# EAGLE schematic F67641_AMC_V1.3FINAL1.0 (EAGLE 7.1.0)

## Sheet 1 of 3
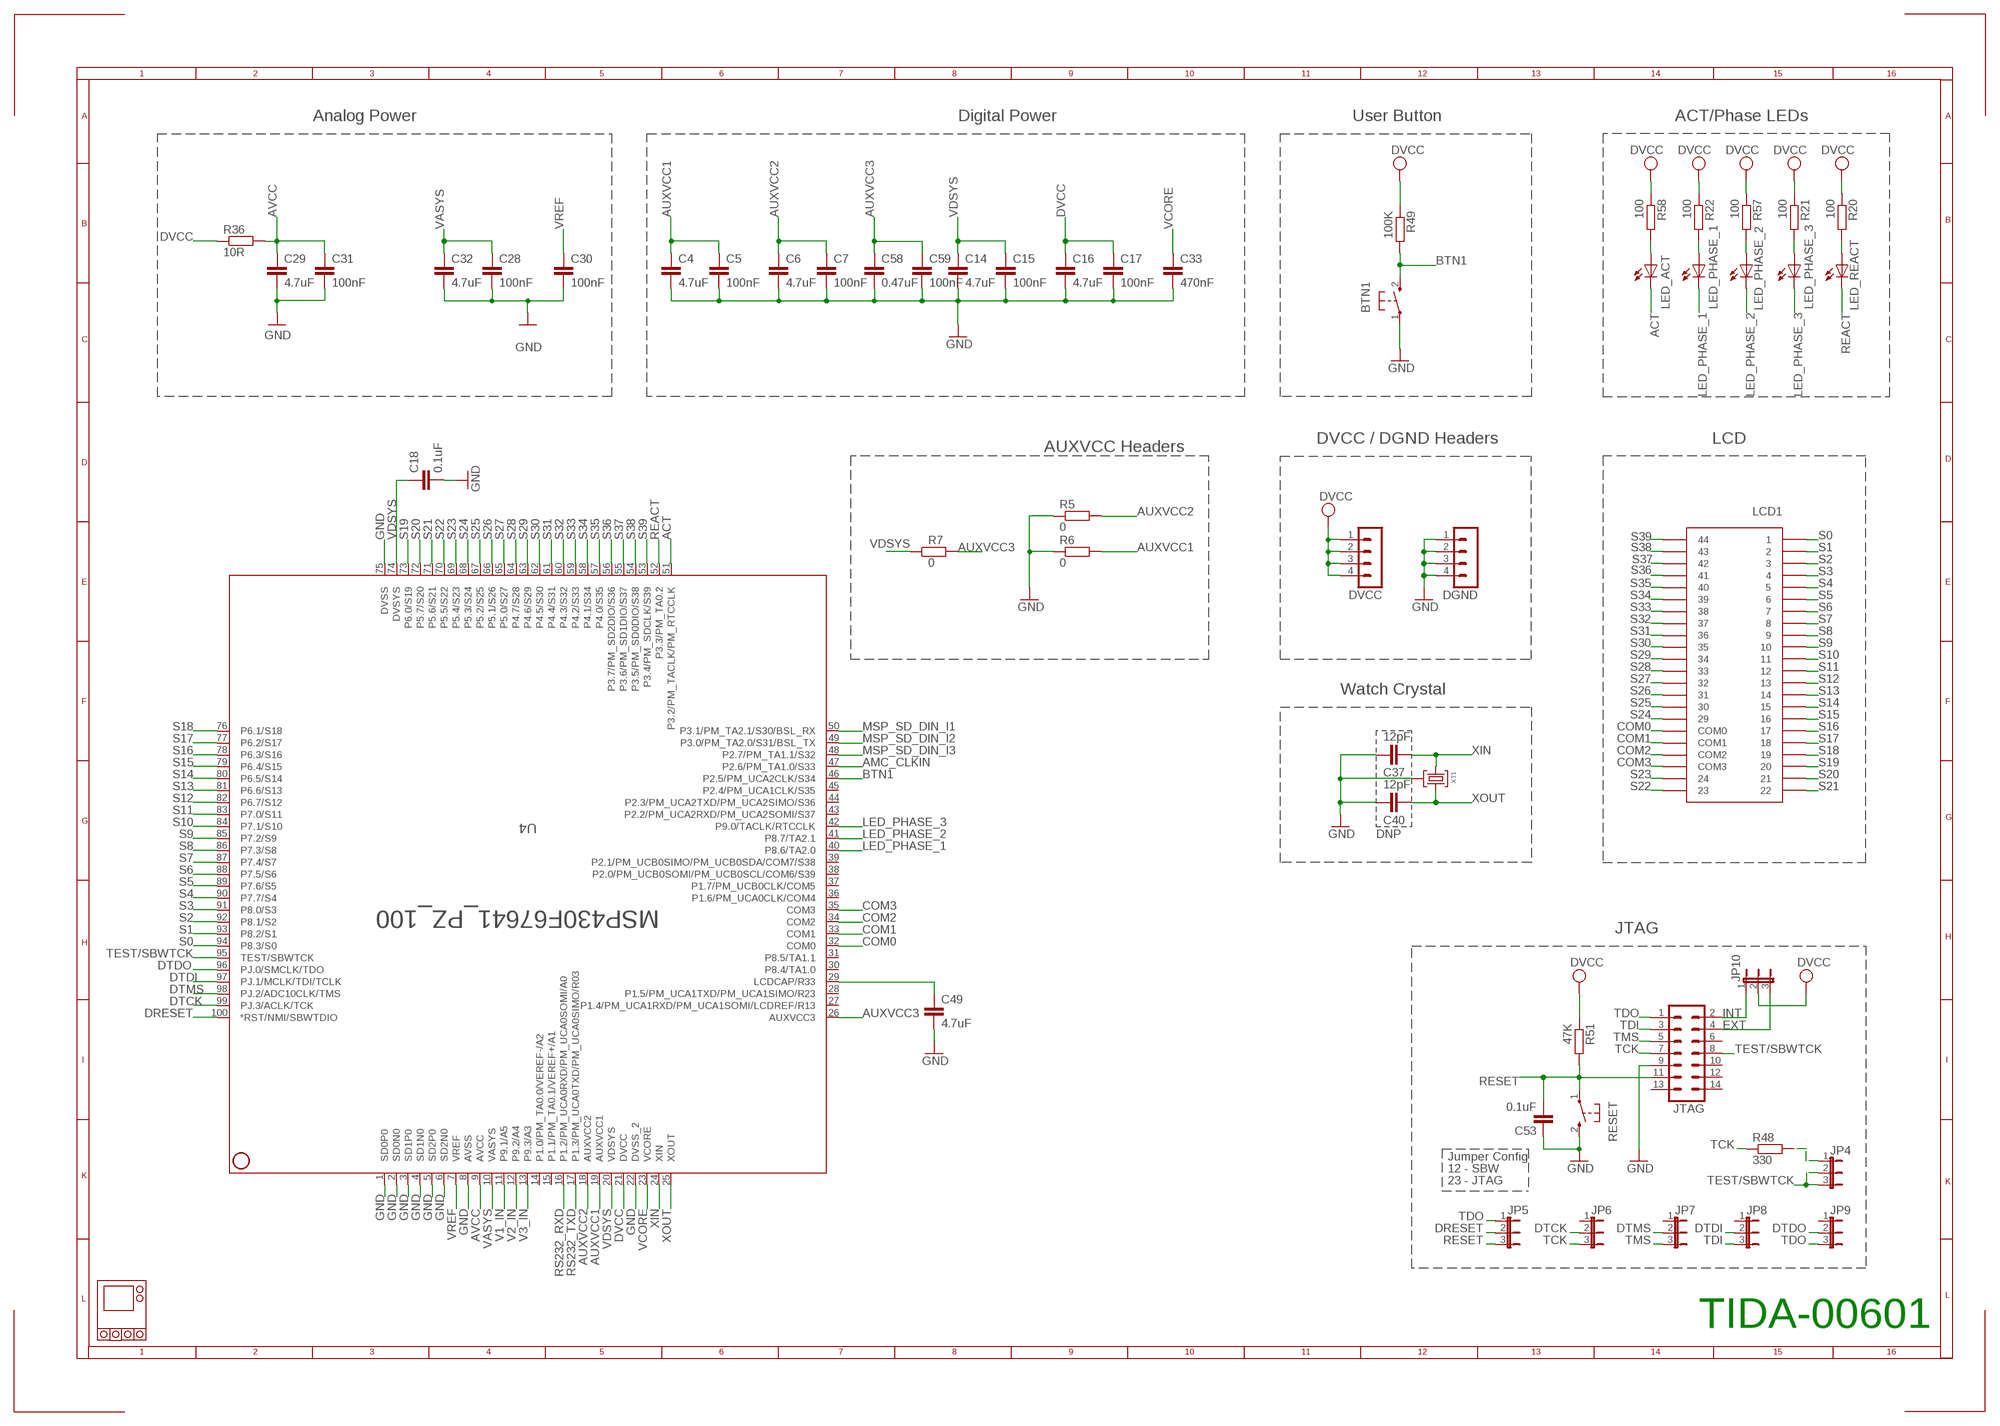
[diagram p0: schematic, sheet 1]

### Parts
BTN1  PB  [PBTH]
C4  4.7uF  C-EUC0603  [C0603]
C5  100nF  C-EUC0603  [C0603]
C6  4.7uF  C-EUC0603  [C0603]
C7  100nF  C-EUC0603  [C0603]
C14  4.7uF  C-EUC0603  [C0603]
C15  100nF  C-EUC0603  [C0603]
C16  4.7uF  C-EUC0603  [C0603]
C17  100nF  C-EUC0603  [C0603]
C18  0.1uF  C-EUC0603  [C0603]
C28  100nF  C-EUC0603  [C0603]
C29  4.7uF  C-EUC0603  [C0603]
C30  100nF  C-EUC0603  [C0603]
C31  100nF  C-EUC0603  [C0603]
C32  4.7uF  C-EUC0603  [C0603]
C33  470nF  C-EUC0603  [C0603]
C37  12pF  C-EUC0603  [C0603]
C40  12pF  C-EUC0603  [C0603]
C49  4.7uF  C-EUC0603  [C0603]
C53  0.1uF  C-EUC0603  [C0603]
C58  0.47uF  C-EUC0603  [C0603]
C59  100nF  C-EUC0603  [C0603]
CASE1  3_PHASE_CASE  [3_PHASE_CASE]
DGND  MA04-1  [MA04-1]
DVCC  MA04-1  [MA04-1]
JP4  JP2E  [JP2]
JP5  JP2E  [JP2]
JP6  JP2E  [JP2]
JP7  JP2E  [JP2]
JP8  JP2E  [JP2]
JP9  JP2E  [JP2]
JP10  JP2E  [JP2]
JTAG  ML14  [ML14]
LCD1  TI_160SEG_LCD  [TI_160SEG_LCD]
LED_ACT  LED3MM  [LED3MM]
LED_PHASE_1  LED3MM  [LED3MM]
LED_PHASE_2  LED3MM  [LED3MM]
LED_PHASE_3  LED3MM  [LED3MM]
LED_REACT  LED3MM  [LED3MM]
R5  0  R-EU_R0603  [R0603]
R6  0  R-EU_R0603  [R0603]
R7  0  R-EU_R0603  [R0603]
R20  100  R-EU_R0603  [R0603]
R21  100  R-EU_R0603  [R0603]
R22  100  R-EU_R0603  [R0603]
R36  10R  R-EU_R0805  [R0805]
R48  330  R-EU_R0603  [R0603]
R49  100K  R-EU_R0603  [R0603]
R51  47K  R-EU_R0603  [R0603]
R57  100  R-EU_R0603  [R0603]
R58  100  R-EU_R0603  [R0603]
RESET  PB  [PBTH]
U4  MSP430F67641_PZ_100  [PZ100]
XT1  CM200T  [CM200T]

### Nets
ACT: LED_ACT.K(C) U4.51(P3.2/PM_TACLK/PM_RTCCLK) ; also sheet 2
AMC_CLKIN: U4.47(P2.6/PM_TA1.0/S33) ; also sheet 3
AUXVCC1: C4.1 C5.1 R6.2 U4.19(AUXVCC1)
AUXVCC2: C6.1 C7.1 R5.2 U4.18(AUXVCC2)
AUXVCC3: C58.1 C59.1 R7.2 U4.26(AUXVCC3)
AVCC: C29.1 C31.1 R36.2 U4.9(AVCC) ; also sheet 2
BTN1: BTN1.2(S) R49.2 U4.46(P2.5/PM_UCA2CLK/S34)
COM0: LCD1.COM0 U4.32(COM0)
COM1: LCD1.COM1 U4.33(COM1)
COM2: LCD1.COM2 U4.34(COM2)
COM3: LCD1.COM3 U4.35(COM3)
DRESET: JP5.2 U4.100(*RST/NMI/SBWTDIO)
DTCK: JP6.2 U4.99(PJ.3/ACLK/TCK)
DTDI: JP8.2 U4.97(PJ.1/MCLK/TDI/TCLK)
DTDO: JP9.2 U4.96(PJ.0/SMCLK/TDO)
DTMS: JP7.2 U4.98(PJ.2/ADC10CLK/TMS)
DVCC: C16.1 C17.1 DVCC.1 DVCC.2 DVCC.3 DVCC.4 JP10.2 R20.1 R21.1 R22.1 R36.1 R49.1 R51.1 R57.1 R58.1 U4.21(DVCC) ; also sheet 2,3
EXT: JP10.3 JTAG.4
GND: BTN1.1(P) C4.2 C5.2 C6.2 C7.2 C14.2 C15.2 C16.2 C17.2 C18.2 C28.2 C29.2 C30.2 C31.2 C32.2 C33.2 C37.2 C40.2 C49.2 C53.1 C58.2 C59.2 DGND.1 DGND.2 DGND.3 DGND.4 JTAG.9 R5.1 R6.1 RESET.2(S) U4.1(SD0P0) U4.2(SD0N0) U4.3(SD1P0) U4.4(SD1N0) U4.5(SD2P0) U4.6(SD2N0) U4.8(AVSS) U4.22(DVSS_2) U4.75(DVSS) XT1.P3 ; also sheet 2,3
INT: JP10.1 JTAG.2
LED_PHASE_1: LED_PHASE_1.K(C) U4.40(P8.6/TA2.0)
LED_PHASE_2: LED_PHASE_2.K(C) U4.41(P8.7/TA2.1)
LED_PHASE_3: LED_PHASE_3.K(C) U4.42(P9.0/TACLK/RTCCLK)
MSP_SD_DIN_I1: U4.50(P3.1/PM_TA2.1/S30/BSL_RX) ; also sheet 3
MSP_SD_DIN_I2: U4.49(P3.0/PM_TA2.0/S31/BSL_TX) ; also sheet 3
MSP_SD_DIN_I3: U4.48(P2.7/PM_TA1.1/S32) ; also sheet 3
N$4: C49.1 U4.29(LCDCAP/R33)
N$5: LED_REACT.A R20.2
N$6: LED_PHASE_3.A R21.2
N$7: LED_PHASE_1.A R22.2
N$34: JP4.1 R48.2
N$44: LED_ACT.A R58.2
N$46: LED_PHASE_2.A R57.2
REACT: LED_REACT.K(C) U4.52(P3.3/PM_TA0.2) ; also sheet 2
RESET: C53.2 JP5.3 JTAG.11 R51.2 RESET.1(P)
RS232_RXD: U4.16(P1.2/PM_UCA0RXD/PM_UCA0SOMI/A0) ; also sheet 2
RS232_TXD: U4.17(P1.3/PM_UCA0TXD/PM_UCA0SIMO/R03) ; also sheet 2
S0: LCD1.1 U4.94(P8.3/S0)
S1: LCD1.2 U4.93(P8.2/S1)
S2: LCD1.3 U4.92(P8.1/S2)
S3: LCD1.4 U4.91(P8.0/S3)
S4: LCD1.5 U4.90(P7.7/S4)
S5: LCD1.6 U4.89(P7.6/S5)
S6: LCD1.7 U4.88(P7.5/S6)
S7: LCD1.8 U4.87(P7.4/S7)
S8: LCD1.9 U4.86(P7.3/S8)
S9: LCD1.10 U4.85(P7.2/S9)
S10: LCD1.11 U4.84(P7.1/S10)
S11: LCD1.12 U4.83(P7.0/S11)
S12: LCD1.13 U4.82(P6.7/S12)
S13: LCD1.14 U4.81(P6.6/S13)
S14: LCD1.15 U4.80(P6.5/S14)
S15: LCD1.16 U4.79(P6.4/S15)
S16: LCD1.17 U4.78(P6.3/S16)
S17: LCD1.18 U4.77(P6.2/S17)
S18: LCD1.19 U4.76(P6.1/S18)
S19: LCD1.20 U4.73(P6.0/S19)
S20: LCD1.21 U4.72(P5.7/S20)
S21: LCD1.22 U4.71(P5.6/S21)
S22: LCD1.23 U4.70(P5.5/S22)
S23: LCD1.24 U4.69(P5.4/S23)
S24: LCD1.29 U4.68(P5.3/S24)
S25: LCD1.30 U4.67(P5.2/S25)
S26: LCD1.31 U4.66(P5.1/S26)
S27: LCD1.32 U4.65(P5.0/S27)
S28: LCD1.33 U4.64(P4.7/S28)
S29: LCD1.34 U4.63(P4.6/S29)
S30: LCD1.35 U4.62(P4.5/S30)
S31: LCD1.36 U4.61(P4.4/S31)
S32: LCD1.37 U4.60(P4.3/S32)
S33: LCD1.38 U4.59(P4.2/S33)
S34: LCD1.39 U4.58(P4.1/S34)
S35: LCD1.40 U4.57(P4.0/S35)
S36: LCD1.41 U4.56(P3.7/PM_SD2DIO/S36)
S37: LCD1.42 U4.55(P3.6/PM_SD1DIO/S37)
S38: LCD1.43 U4.54(P3.5/PM_SD0DIO/S38)
S39: LCD1.44 U4.53(P3.4/PM_SDCLK/S39)
TCK: JP6.3 JTAG.7 R48.1
TDI: JP8.3 JTAG.3
TDO: JP5.1 JP9.3 JTAG.1
TEST/SBWTCK: JP4.2 JP4.3 JTAG.8 U4.95(TEST/SBWTCK)
TMS: JP7.3 JTAG.5
V1_IN: U4.11(P9.1/A5) ; also sheet 2
V2_IN: U4.12(P9.2/A4) ; also sheet 2
V3_IN: U4.13(P9.3/A3) ; also sheet 2
VASYS: C28.1 C32.1 U4.10(VASYS)
VCORE: C33.1 U4.23(VCORE)
VDSYS: C14.1 C15.1 C18.1 R7.1 U4.20(VDSYS) U4.74(DVSYS)
VREF: C30.1 U4.7(VREF)
XIN: C37.1 U4.24(XIN) XT1.P2
XOUT: C40.1 U4.25(XOUT) XT1.P1
Unconnected: JP6.1 JP7.1 JP8.1 JP9.1 JTAG.6 JTAG.10 JTAG.12 JTAG.13 JTAG.14 U4.14(P1.0/PM_TA0.0/VEREF-/A2) U4.15(P1.1/PM_TA0.1/VEREF+/A1) U4.27(P1.4/PM_UCA1RXD/PM_UCA1SOMI/LCDREF/R13) U4.28(P1.5/PM_UCA1TXD/PM_UCA1SIMO/R23) U4.30(P8.4/TA1.0) U4.31(P8.5/TA1.1) U4.36(P1.6/PM_UCA0CLK/COM4) U4.37(P1.7/PM_UCB0CLK/COM5) U4.38(P2.0/PM_UCB0SOMI/PM_UCB0SCL/COM6/S39) U4.39(P2.1/PM_UCB0SIMO/PM_UCB0SDA/COM7/S38) U4.43(P2.2/PM_UCA2RXD/PM_UCA2SOMI/S37) U4.44(P2.3/PM_UCA2TXD/PM_UCA2SIMO/S36) U4.45(P2.4/PM_UCA1CLK/S35)

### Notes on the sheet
- Analog Power | Digital Power | User Button | ACT/Phase LEDs
- DVCC / DGND Headers | LCD
- AUXVCC Headers
- Watch Crystal
- DNP
- JTAG
- Jumper Config
- 12 - SBW
- 23 - JTAG
- TIDA-00601

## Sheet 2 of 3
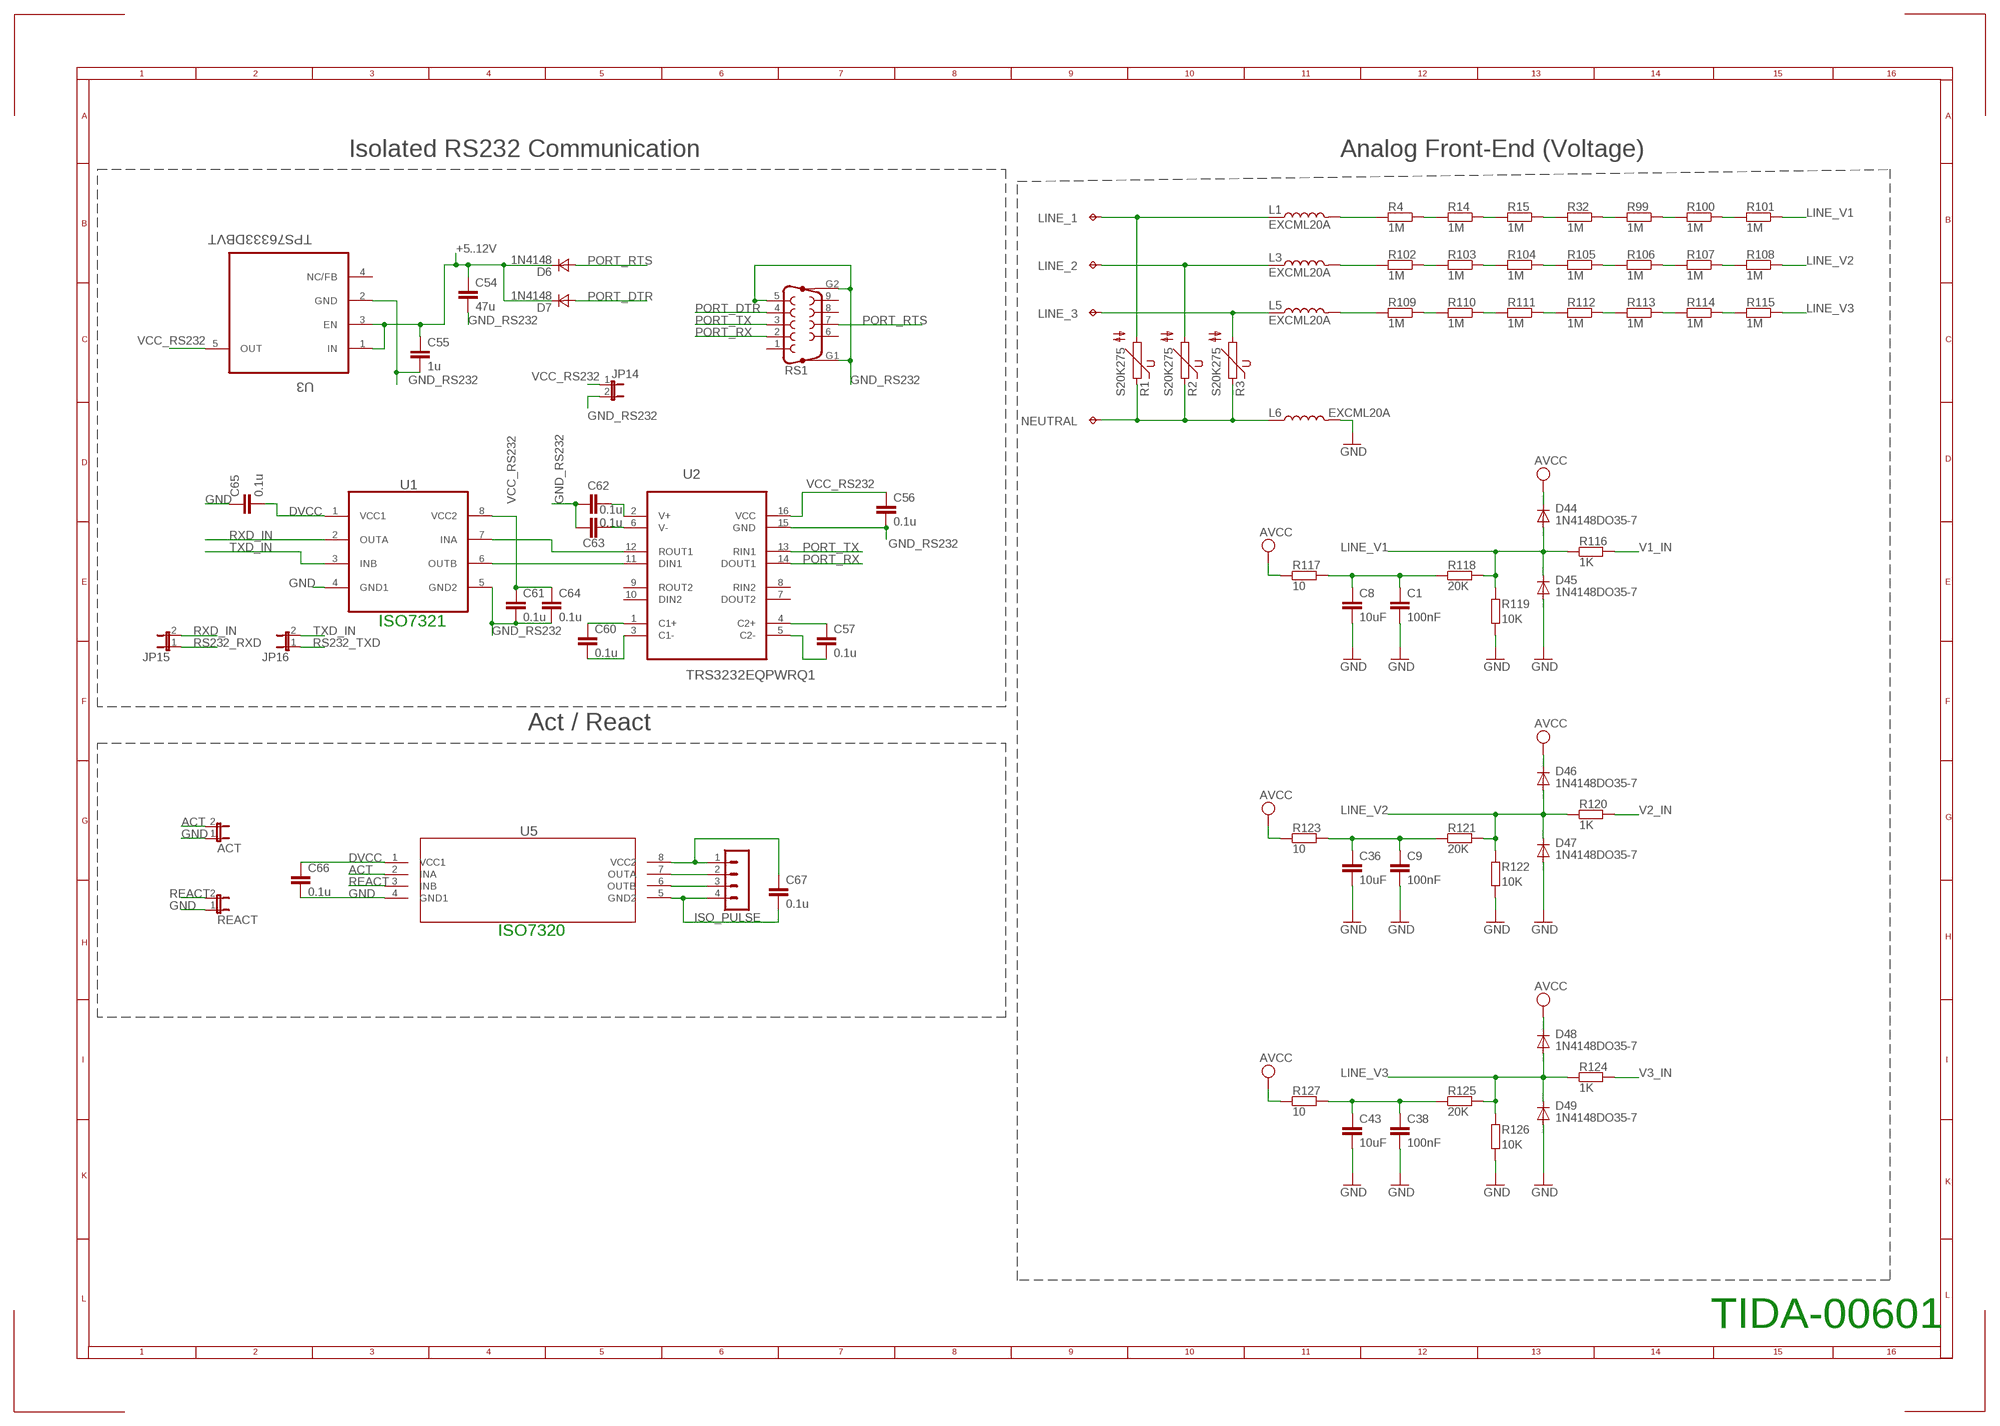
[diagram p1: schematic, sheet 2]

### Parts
ACT  JP1E  [JP1]
C1  100nF  C-EUC0805  [C0805]
C8  10uF  C-EUC0805  [C0805]
C9  100nF  C-EUC0805  [C0805]
C36  10uF  C-EUC0805  [C0805]
C38  100nF  C-EUC0805  [C0805]
C43  10uF  C-EUC0805  [C0805]
C54  47u  C-EUC1206K  [C1206K]
C55  1u  C-EUC0603  [C0603]
C56  0.1u  C-EUC0603  [C0603]
C57  0.1u  C-EUC0603  [C0603]
C60  0.1u  C-EUC0603  [C0603]
C61  0.1u  C-EUC0603  [C0603]
C62  0.1u  C-EUC0603  [C0603]
C63  0.1u  C-EUC0603  [C0603]
C64  0.1u  C-EUC0603  [C0603]
C65  0.1u  C-EUC0603  [C0603]
C66  0.1u  C-EUC0603  [C0603]
C67  0.1u  C-EUC0603  [C0603]
D6  1N4148  DSOD323  [SOD323]
D7  1N4148  DSOD323  [SOD323]
D44  1N4148DO35-7  DIODE-SOD523  [SOD523]
D45  1N4148DO35-7  DIODE-SOD523  [SOD523]
D46  1N4148DO35-7  DIODE-SOD523  [SOD523]
D47  1N4148DO35-7  DIODE-SOD523  [SOD523]
D48  1N4148DO35-7  DIODE-SOD523  [SOD523]
D49  1N4148DO35-7  DIODE-SOD523  [SOD523]
ISO_PULSE  MA04-1  [MA04-1]
JP14  JP1E  [JP1]
JP15  JP1E  [JP1]
JP16  JP1E  [JP1]
L1  EXCML20A  EXCELSA390805  [R0805]
L3  EXCML20A  EXCELSA390805  [R0805]
L5  EXCML20A  EXCELSA390805  [R0805]
L6  EXCML20A  EXCELSA390805  [R0805]
LINE_1  TPPAD1-20  [P1-20]
LINE_2  TPPAD1-20  [P1-20]
LINE_3  TPPAD1-20  [P1-20]
NEUTRAL  TPPAD1-20  [P1-20]
R1  S20K275  [S20K275]
R2  S20K275  [S20K275]
R3  S20K275  [S20K275]
R4  1M  R-EU_R0805  [R0805]
R14  1M  R-EU_R0805  [R0805]
R15  1M  R-EU_R0805  [R0805]
R32  1M  R-EU_R0805  [R0805]
R99  1M  R-EU_R0805  [R0805]
R100  1M  R-EU_R0805  [R0805]
R101  1M  R-EU_R0805  [R0805]
R102  1M  R-EU_R0805  [R0805]
R103  1M  R-EU_R0805  [R0805]
R104  1M  R-EU_R0805  [R0805]
R105  1M  R-EU_R0805  [R0805]
R106  1M  R-EU_R0805  [R0805]
R107  1M  R-EU_R0805  [R0805]
R108  1M  R-EU_R0805  [R0805]
R109  1M  R-EU_R0805  [R0805]
R110  1M  R-EU_R0805  [R0805]
R111  1M  R-EU_R0805  [R0805]
R112  1M  R-EU_R0805  [R0805]
R113  1M  R-EU_R0805  [R0805]
R114  1M  R-EU_R0805  [R0805]
R115  1M  R-EU_R0805  [R0805]
R116  1K  R-EU_R0805  [R0805]
R117  10  R-EU_R0805  [R0805]
R118  20K  R-EU_R0805  [R0805]
R119  10K  R-EU_R0805  [R0805]
R120  1K  R-EU_R0805  [R0805]
R121  20K  R-EU_R0805  [R0805]
R122  10K  R-EU_R0805  [R0805]
R123  10  R-EU_R0805  [R0805]
R124  1K  R-EU_R0805  [R0805]
R125  20K  R-EU_R0805  [R0805]
R126  10K  R-EU_R0805  [R0805]
R127  10  R-EU_R0805  [R0805]
REACT  JP1E  [JP1]
RS1  F09VP  [F09VP]
U1  ISO7421D  [SOIC127P600X175-8N]
U2  TRS3232EQPWRQ1  [SOP65P640X120-16N]
U3  TPS76333DBVT  [SOT95P280X145-5N]
U5  ISO7420_D_8  [D8]

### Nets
+5..12V: C54.1 C55.1 D6.1(C) D7.1(C) U3.1(IN) U3.3(EN)
ACT: ACT.2 U5.2(INA) ; also sheet 1
AVCC: D44.C D46.C D48.C R117.1 R123.1 R127.1 ; also sheet 1
DVCC: C65.2 C66.1 U1.1(VCC1) U5.1(VCC1) ; also sheet 1,3
GND: ACT.1 C1.2 C8.2 C9.2 C36.2 C38.2 C43.2 C65.1 C66.2 D45.A D47.A D49.A L6.2 R119.1 R122.1 R126.1 REACT.1 U1.4(GND1) U5.4(GND1) ; also sheet 1,3
GND_RS232: C54.2 C55.2 C56.2 C61.2 C62.1 C63.1 C64.2 JP14.2 RS1.5 RS1.G1 RS1.G2 U1.5(GND2) U2.15(GND) U3.2(GND)
LINE_1: L1.1 LINE_1.TP R1.2
LINE_2: L3.1 LINE_2.TP R2.2
LINE_3: L5.1 LINE_3.TP R3.2
LINE_V1: D44.A D45.C R101.1 R116.1 R118.2 R119.2
LINE_V2: D46.A D47.C R108.1 R120.1 R121.2 R122.2
LINE_V3: D48.A D49.C R115.1 R124.1 R125.2 R126.2
N$3: C67.1 ISO_PULSE.1 U5.8(VCC2)
N$9: C57.1 U2.4(C2+)
N$11: ISO_PULSE.2 U5.7(OUTA)
N$12: ISO_PULSE.3 U5.6(OUTB)
N$22: C57.2 U2.5(C2-)
N$24: C60.1 U2.1(C1+)
N$26: C60.2 U2.3(C1-)
N$28: U1.7(INA) U2.12(ROUT1)
N$33: U1.6(OUTB) U2.11(DIN1)
N$36: C62.2 U2.2(V+)
N$40: C63.2 U2.6(V-)
N$43: C67.2 ISO_PULSE.4 U5.5(GND2)
N$96: R4.1 R14.2
N$97: R14.1 R15.2
N$98: R15.1 R32.2
N$99: R32.1 R99.2
N$100: R99.1 R100.2
N$101: R100.1 R101.2
N$102: R102.1 R103.2
N$103: R103.1 R104.2
N$104: R104.1 R105.2
N$105: R105.1 R106.2
N$106: R106.1 R107.2
N$107: R107.1 R108.2
N$108: R109.1 R110.2
N$109: R110.1 R111.2
N$110: R111.1 R112.2
N$111: R112.1 R113.2
N$112: R113.1 R114.2
N$113: R114.1 R115.2
N$114: L1.2 R4.2
N$115: L3.2 R102.2
N$116: L5.2 R109.2
N$117: C9.1 C36.1 R121.1 R123.2
N$118: C1.1 C8.1 R117.2 R118.1
N$119: C38.1 C43.1 R125.1 R127.2
NEUTRAL: L6.1 NEUTRAL.TP R1.1 R2.1 R3.1
PORT_DTR: D7.2(A) RS1.4
PORT_RTS: D6.2(A) RS1.7
PORT_RX: RS1.2 U2.14(DOUT1)
PORT_TX: RS1.3 U2.13(RIN1)
REACT: REACT.2 U5.3(INB) ; also sheet 1
RS232_RXD: JP15.1 ; also sheet 1
RS232_TXD: JP16.1 ; also sheet 1
RXD_IN: JP15.2 U1.2(OUTA)
TXD_IN: JP16.2 U1.3(INB)
V1_IN: R116.2 ; also sheet 1
V2_IN: R120.2 ; also sheet 1
V3_IN: R124.2 ; also sheet 1
VCC_RS232: C56.1 C61.1 C64.1 JP14.1 U1.8(VCC2) U2.16(VCC) U3.5(OUT)
Unconnected: RS1.1 RS1.6 RS1.8 RS1.9 U2.7(DOUT2) U2.8(RIN2) U2.9(ROUT2) U2.10(DIN2) U3.4(NC/FB)

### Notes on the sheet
- Isolated RS232 Communication | Analog Front-End (Voltage)
- ISO7321
- Act / React
- ISO7320
- TIDA-00601

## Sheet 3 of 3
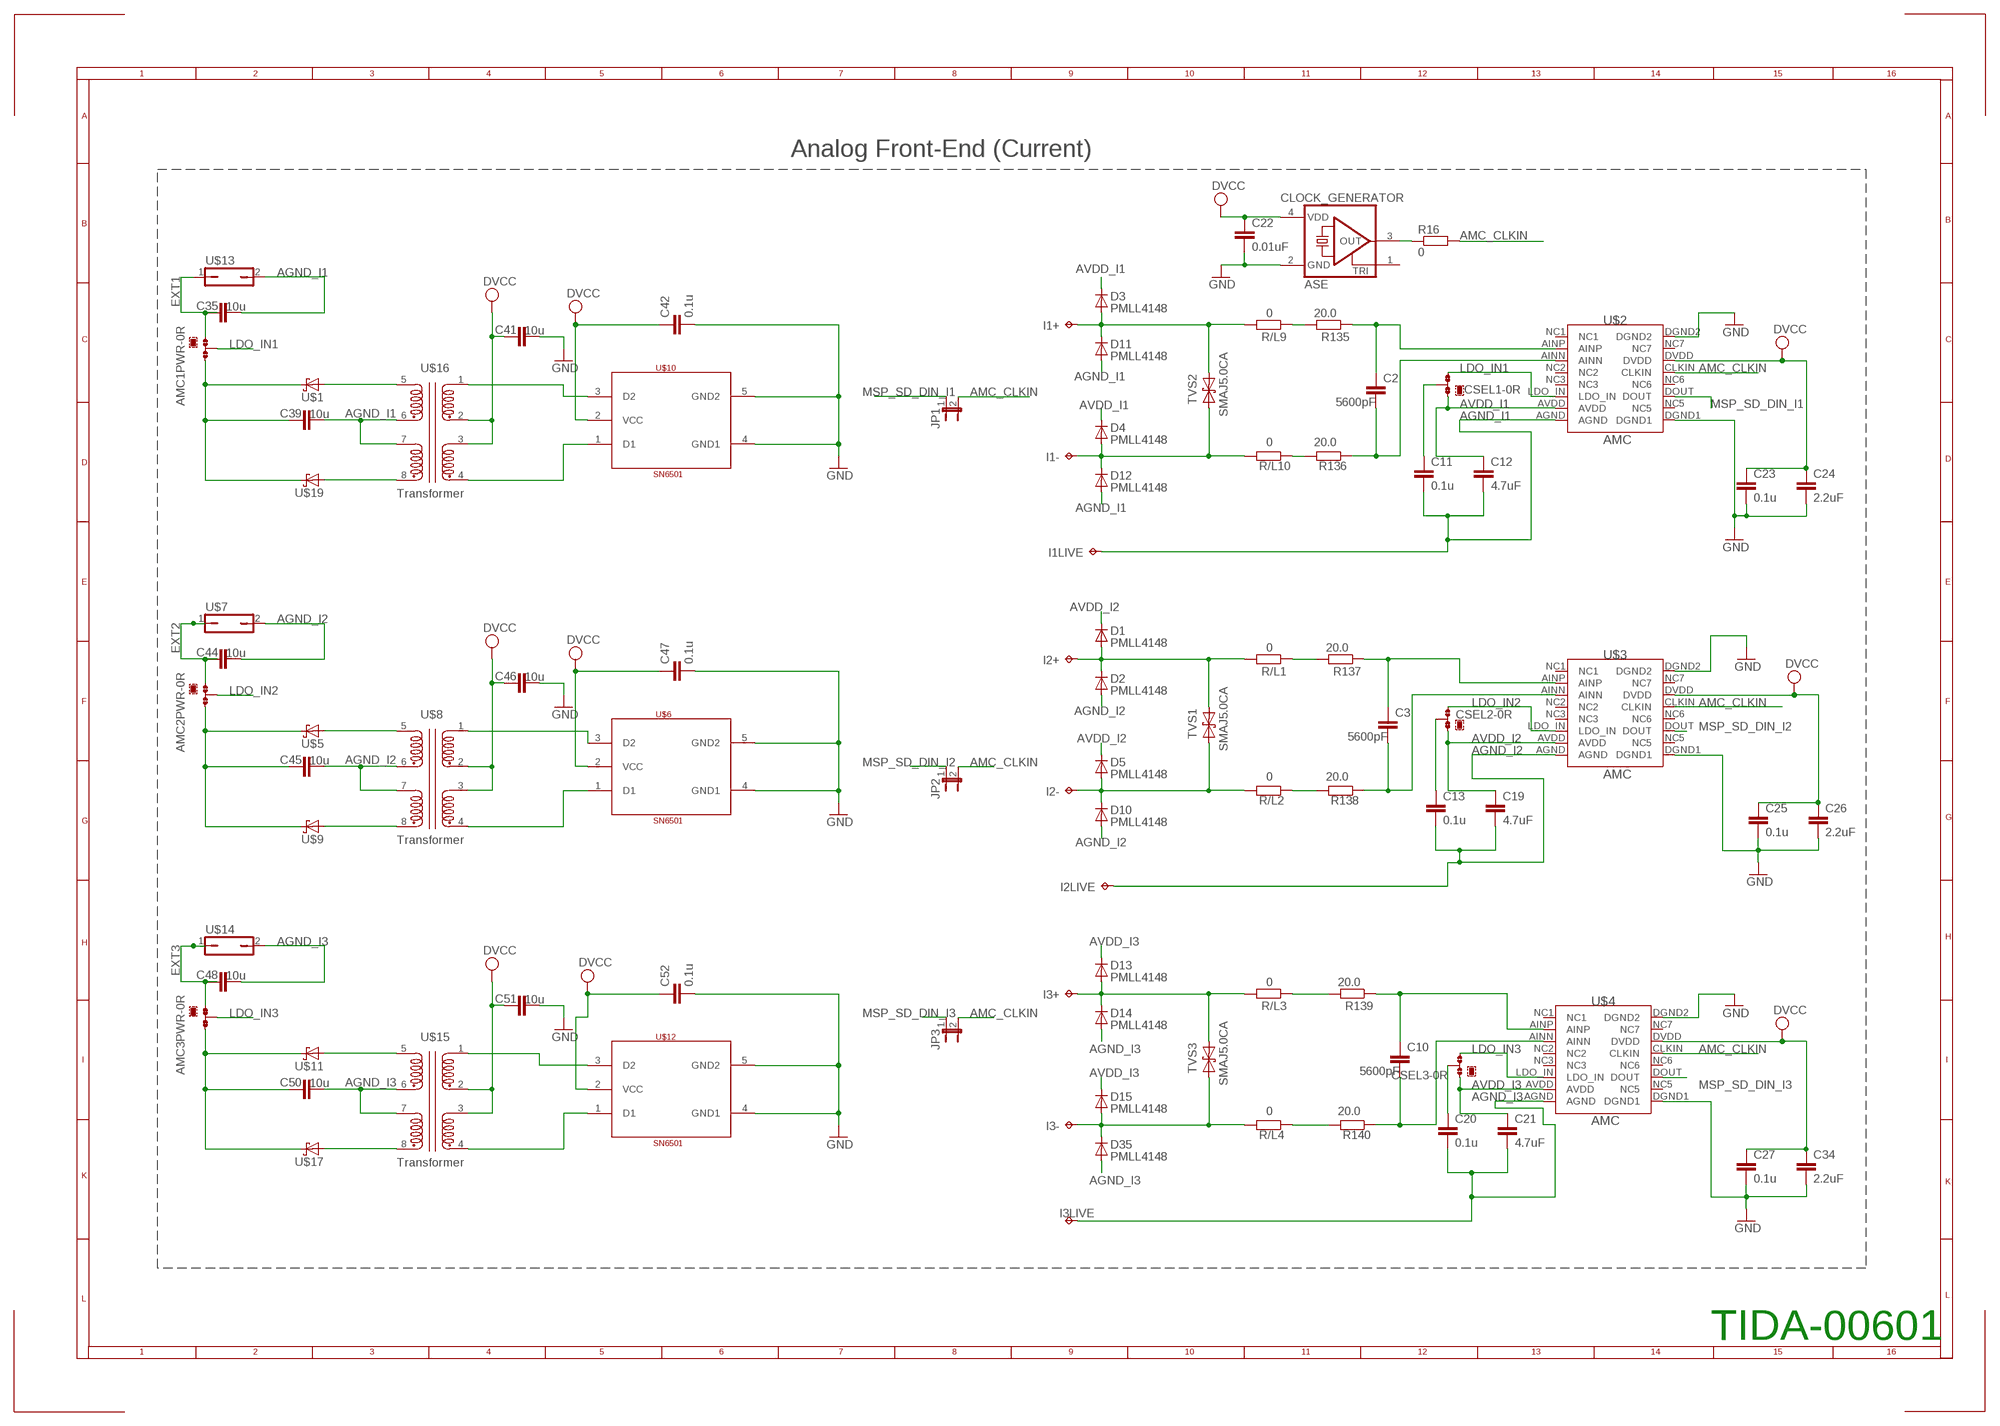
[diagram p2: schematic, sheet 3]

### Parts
AMC1PWR  0R-JUMPA  [A0R-JMP]
AMC2PWR  0R-JUMPA  [A0R-JMP]
AMC3PWR  0R-JUMPA  [A0R-JMP]
C2  5600pF  C-EUC0603  [C0603]
C3  5600pF  C-EUC0603  [C0603]
C10  5600pF  C-EUC0603  [C0603]
C11  0.1u  C-EUC0805  [C0805]
C12  4.7uF  C-EUC0805  [C0805]
C13  0.1u  C-EUC0805  [C0805]
C19  4.7uF  C-EUC0805  [C0805]
C20  0.1u  C-EUC0805  [C0805]
C21  4.7uF  C-EUC0805  [C0805]
C22  0.01uF  C-EUC0603  [C0603]
C23  0.1u  C-EUC0805  [C0805]
C24  2.2uF  C-EUC0805  [C0805]
C25  0.1u  C-EUC0805  [C0805]
C26  2.2uF  C-EUC0805  [C0805]
C27  0.1u  C-EUC0805  [C0805]
C34  2.2uF  C-EUC0805  [C0805]
C35  10u  C-EUC0805  [C0805]
C39  10u  C-EUC0805  [C0805]
C41  10u  C-EUC0805  [C0805]
C42  0.1u  C-EUC0805  [C0805]
C44  10u  C-EUC0805  [C0805]
C45  10u  C-EUC0805  [C0805]
C46  10u  C-EUC0805  [C0805]
C47  0.1u  C-EUC0805  [C0805]
C48  10u  C-EUC0805  [C0805]
C50  10u  C-EUC0805  [C0805]
C51  10u  C-EUC0805  [C0805]
C52  0.1u  C-EUC0805  [C0805]
CLOCK_GENERATOR  ASE  [ASE]
CSEL1  0R-JUMPA  [A0R-JMP]
CSEL2  0R-JUMPA  [A0R-JMP]
CSEL3  0R-JUMPA  [A0R-JMP]
D1  PMLL4148  [SOD80C]
D2  PMLL4148  [SOD80C]
D3  PMLL4148  [SOD80C]
D4  PMLL4148  [SOD80C]
D5  PMLL4148  [SOD80C]
D10  PMLL4148  [SOD80C]
D11  PMLL4148  [SOD80C]
D12  PMLL4148  [SOD80C]
D13  PMLL4148  [SOD80C]
D14  PMLL4148  [SOD80C]
D15  PMLL4148  [SOD80C]
D35  PMLL4148  [SOD80C]
I1+  TPPAD1-20  [P1-20]
I1-  TPPAD1-20  [P1-20]
I1LIVE  TPPAD1-20  [P1-20]
I2+  TPPAD1-20  [P1-20]
I2-  TPPAD1-20  [P1-20]
I2LIVE  TPPAD1-20  [P1-20]
I3+  TPPAD1-20  [P1-20]
I3-  TPPAD1-20  [P1-20]
I3LIVE  TPPAD1-20  [P1-20]
JP1  JP1E  [JP1]
JP2  JP1E  [JP1]
JP3  JP1E  [JP1]
R16  0  R-EU_R0603  [R0603]
R135  20.0  R-EU_R0603  [R0603]
R136  20.0  R-EU_R0603  [R0603]
R137  20.0  R-EU_R0603  [R0603]
R138  20.0  R-EU_R0603  [R0603]
R139  20.0  R-EU_R0603  [R0603]
R140  20.0  R-EU_R0603  [R0603]
R/L1  0  R-EU_R0603  [R0603]
R/L2  0  R-EU_R0603  [R0603]
R/L3  0  R-EU_R0603  [R0603]
R/L4  0  R-EU_R0603  [R0603]
R/L9  0  R-EU_R0603  [R0603]
R/L10  0  R-EU_R0603  [R0603]
TVS1  SMAJ5.0CA  [DO214AC]
TVS2  SMAJ5.0CA  [DO214AC]
TVS3  SMAJ5.0CA  [DO214AC]
U$1  DIODE-SCHOTTKY-CUSTOM  [SOD123]
U$2  AMC  [SOIC-16DW]
U$3  AMC  [SOIC-16DW]
U$4  AMC  [SOIC-16DW]
U$5  DIODE-SCHOTTKY-CUSTOM  [SOD123]
U$6  SN6501  [SOT23-DBV]
U$7  CUSTOM_TERMINAL_BLOCK  [TERMINALBLOCK5.08]
U$8  CUSTOM_TRANSFORMER_AMC  [DA2303-AL]
U$9  DIODE-SCHOTTKY-CUSTOM  [SOD123]
U$10  SN6501  [SOT23-DBV]
U$11  DIODE-SCHOTTKY-CUSTOM  [SOD123]
U$12  SN6501  [SOT23-DBV]
U$13  CUSTOM_TERMINAL_BLOCK  [TERMINALBLOCK5.08]
U$14  CUSTOM_TERMINAL_BLOCK  [TERMINALBLOCK5.08]
U$15  CUSTOM_TRANSFORMER_AMC  [DA2303-AL]
U$16  CUSTOM_TRANSFORMER_AMC  [DA2303-AL]
U$17  DIODE-SCHOTTKY-CUSTOM  [SOD123]
U$19  DIODE-SCHOTTKY-CUSTOM  [SOD123]

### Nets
AGND_I1: C11.2 C12.2 C35.2 C39.2 D11.A D12.A I1LIVE.TP U$2.AGND U$13.2 U$16.6 U$16.7
AGND_I2: C13.2 C19.2 C44.2 C45.2 D2.A D10.A I2LIVE.TP U$3.AGND U$7.2 U$8.6 U$8.7
AGND_I3: C20.2 C21.2 C48.2 C50.2 D14.A D35.A I3LIVE.TP U$4.AGND U$14.2 U$15.6 U$15.7
AMC_CLKIN: JP1.2 JP2.2 JP3.2 R16.2 U$2.CLKIN U$3.CLKIN U$4.CLKIN ; also sheet 1
AVDD_I1: C12.1 CSEL1.1 D3.C D4.C U$2.AVDD
AVDD_I2: C19.1 CSEL2.1 D1.C D5.C U$3.AVDD
AVDD_I3: C21.1 CSEL3.1 D13.C D15.C U$4.AVDD
CUR1+: D3.A D11.C I1+.TP R/L9.2 TVS2.C(K)
CUR1+1: D1.A D2.C I2+.TP R/L1.2 TVS1.C(K)
CUR1+2: D13.A D14.C I3+.TP R/L3.2 TVS3.C(K)
CUR1-: D4.A D12.C I1-.TP R/L10.2 TVS2.A
CUR1-1: D5.A D10.C I2-.TP R/L2.2 TVS1.A
CUR1-2: D15.A D35.C I3-.TP R/L4.2 TVS3.A
DVCC: C22.1 C23.1 C24.1 C25.1 C26.1 C27.1 C34.1 C41.1 C42.1 C46.1 C47.1 C51.1 C52.1 CLOCK_GENERATOR.4(VDD) U$2.DVDD U$3.DVDD U$4.DVDD U$6.2(VCC) U$8.2 U$8.3 U$10.2(VCC) U$12.2(VCC) U$15.2 U$15.3 U$16.2 U$16.3 ; also sheet 1,2
EXT1: AMC1PWR.1 C35.1 U$13.1
EXT2: AMC2PWR.1 C44.1 U$7.1
EXT3: AMC3PWR.1 C48.1 U$14.1
GND: C22.2 C23.2 C24.2 C25.2 C26.2 C27.2 C34.2 C41.2 C42.2 C46.2 C47.2 C51.2 C52.2 CLOCK_GENERATOR.2(GND) U$2.DGND1 U$2.DGND2 U$3.DGND1 U$3.DGND2 U$4.DGND1 U$4.DGND2 U$6.4(GND1) U$6.5(GND2) U$10.4(GND1) U$10.5(GND2) U$12.4(GND1) U$12.5(GND2) ; also sheet 1,2
LDO_IN1: AMC1PWR.2 CSEL1.3 U$2.LDO_IN
LDO_IN2: AMC2PWR.2 CSEL2.3 U$3.LDO_IN
LDO_IN3: AMC3PWR.2 CSEL3.3 U$4.LDO_IN
MSP_SD_DIN_I1: JP1.1 U$2.DOUT ; also sheet 1
MSP_SD_DIN_I2: JP2.1 U$3.DOUT ; also sheet 1
MSP_SD_DIN_I3: JP3.1 U$4.DOUT ; also sheet 1
N$1: C11.1 CSEL1.2
N$2: AMC1PWR.3 C39.1 U$1.C U$19.C
N$8: R135.2 R/L9.1
N$13: R136.2 R/L10.1
N$14: C2.1 R135.1 U$2.AINP
N$15: C2.2 R136.1 U$2.AINN
N$16: R137.2 R/L1.1
N$17: AMC2PWR.3 C45.1 U$5.C U$9.C
N$18: C13.1 CSEL2.2
N$19: R138.2 R/L2.1
N$20: C3.1 R137.1 U$3.AINP
N$21: C3.2 R138.1 U$3.AINN
N$23: R139.2 R/L3.1
N$25: R140.2 R/L4.1
N$27: C10.1 R139.1 U$4.AINP
N$29: C10.2 R140.1 U$4.AINN
N$30: C20.1 CSEL3.2
N$31: CLOCK_GENERATOR.3(OUT) R16.1
N$32: U$1.A U$16.5
N$35: U$16.8 U$19.A
N$37: U$5.A U$8.5
N$38: U$10.1(D1) U$16.4
N$39: U$10.3(D2) U$16.1
N$42: U$8.8 U$9.A
N$45: U$6.1(D1) U$8.4
N$47: U$6.3(D2) U$8.1
N$48: AMC3PWR.3 C50.1 U$11.C U$17.C
N$49: U$11.A U$15.5
N$50: U$15.8 U$17.A
N$51: U$12.1(D1) U$15.4
N$52: U$12.3(D2) U$15.1
Unconnected: CLOCK_GENERATOR.1(TRI) U$2.NC1 U$2.NC2 U$2.NC3 U$2.NC5 U$2.NC6 U$2.NC7 U$3.NC1 U$3.NC2 U$3.NC3 U$3.NC5 U$3.NC6 U$3.NC7 U$4.NC1 U$4.NC2 U$4.NC3 U$4.NC5 U$4.NC6 U$4.NC7

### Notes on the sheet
- Analog Front-End (Current)
- TIDA-00601

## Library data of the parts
ACT JP1-JP3 REACT = custom_jumper:JP1E: JUMPER
AMC1PWR AMC2PWR AMC3PWR CSEL1-CSEL3 = jump-0r-smd:0R-JUMP: SMD 0R 0805 Jumper
BTN1 RESET = electricalmeter:PB: OMRON SWITCH
C1 C8 C9 C11-C13 C19-C21 C23-C27 C34-C36 C38 C39 C41-C48 C50-C52 = rcl:C-EU: CAPACITOR, European symbol
C2-C7 C10 C14-C18 C22 C28-C33 C37 C40 C49 C53 C58 C59 = resistor:C-EU: CAPACITOR, European symbol
C54 = rcl:C-EU: CAPACITOR, European symbol; DIGIKEY: 445-8047-1-ND
C55-C57 C60-C67 = rcl:C-EU: CAPACITOR, European symbol; DIGIKEY: 445-5956-1-ND
CASE1 = meter_cases:3_PHASE_CASE
CLOCK_GENERATOR = crystal:ASE: 3.3Vdc CMOS SMD CRYSTAL CLOCK OSCILLATOR SOurce: www.abracon.com; OC_FARNELL: unknown; OC_NEWARK: unknown
D1-D5 D10-D15 D35 = FE449x EVM:PMLL4148: DIODE
D6 D7 = zetex:D: DIODE; DIGIKEY: 1N4148WSFSCT-ND; MPN: CDSOD323-T05C; OC_FARNELL: 1824860; OC_NEWARK: 79R6078
D44-D49 = diode:DIODE-: DIODE
DGND DVCC ISO_PULSE = custom_con-lstb:MA04-1: PIN HEADER; OC_FARNELL: unknown; OC_NEWARK: unknown
I1+ I1- I1LIVE I2+ I2- I2LIVE I3+ I3- I3LIVE LINE_1-LINE_3 NEUTRAL = testpad:TP: Test pad
JP4-JP10 = custom_jumper:JP2E: JUMPER
JP14-JP16 = jumper:JP1E: JUMPER; DIGIKEY: 609-4434-ND
JTAG = con-ml:ML14: HARTING; OC_FARNELL: unknown; OC_NEWARK: unknown
L1 L3 L5 L6 = FE449x EVM:EXCELSA39: INDUCTOR
LCD1 = Personal:TI_160SEG_LCD
LED_ACT LED_PHASE_1-LED_PHASE_3 LED_REACT = led:LED: LED
R1-R3 = varistor:S20K275: VARISTOR
R4-R7 R14-R16 R20-R22 R32 R48 R49 R51 R57 R58 R99-R127 R135-R140 R/L1-R/L4 R/L9 R/L10 = resistor:R-EU_: RESISTOR, European symbol
R36 = rcl:R-EU_: RESISTOR, European symbol
RS1 = con-subd:F09VP: SUB-D; DIGIKEY: A32119-ND; OC_FARNELL: unknown; OC_NEWARK: unknown
TVS1-TVS3 = FE449x EVM:SMAJ5.0CA
U1 = Texas Instruments_By_element14_Batch_1:ISO7421D: Low-Power Dual Digital Isolators; DIGIKEY: 296-25187-5-ND; MPN: ISO7421D; OC_FARNELL: -; OC_NEWARK: 33R2484; PACKAGE: SOIC-8; SUPPLIER: Texas Instruments
U2 = Texas Instruments_By_element14_Batch_1:TRS3232EQPWRQ1: RS-232 LINE DRIVER/RECEIVER; DIGIKEY: 296-24863-1-ND; MPN: TRS3232EQPWRQ1; OC_FARNELL: -; OC_NEWARK: 09R6724; PACKAGE: TSSOP-16; SUPPLIER: Texas Instruments
U3 = Texas Instruments_By_element14_Batch_1:TPS76333DBVT: Low Power 150mA Low Dropout Linear Regulator; DIGIKEY: 296-11021-1-ND; MPN: TPS76333DBVT; OC_FARNELL: 8461376; OC_NEWARK: 96C8605; PACKAGE: SOT-23-5; SUPPLIER: Texas Instruments
U4 = F67641:MSP430F67641_PZ_100; DATASHEETURL: http://www.ti.com/lit/gpn/MSP430F67641; DESCRIPTION: MSP430F67641 Mixed Signal Microcontroller; FAMILY_NAME: 6 Series with LCD; GENERIC_PART_NUMBER: MSP430F67641; INDUSTRY_STD_PKG_TYPE: LQFP; MANUFACTURER: Texas Instruments; MANUFACTURER_PART_NUMBER: msp430f67641_pz_100; PACKAGE_DESIGNATOR: PZ; PIN_COUNT: 100; VENDOR: Texas Instruments
U5 = TIiso:ISO7420_D_8; DATASHEETURL: http://www.ti.com/lit/gpn/ISO7420; DESCRIPTION: Low Power Dual Channel Isolators; FAMILY_NAME: ISOLATOR; GENERIC_PART_NUMBER: ISO7420; INDUSTRY_STD_PKG_TYPE: SOIC; MANUFACTURER: Texas Instruments; MANUFACTURER_PART_NUMBER: iso7420_d_8; PACKAGE_DESIGNATOR: D; PIN_COUNT: 8; VENDOR: Texas Instruments
U$1 U$5 U$9 U$11 U$17 U$19 = diode:DIODE-SCHOTTKY-CUSTOM: custom SOD123 used in AMC
U$2-U$4 = amc:AMC
U$6 U$10 U$12 = texas:SN6501
U$7 U$13 U$14 = jumper:CUSTOM_TERMINAL_BLOCK
U$8 U$15 U$16 = trafo-bei:CUSTOM_TRANSFORMER_AMC
XT1 = F20xx PIR Demo & Eval:CM200T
